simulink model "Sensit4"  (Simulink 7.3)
settings: Solver=ode45  StartTime=0.0  StopTime=10.0  RelTol=1e-3
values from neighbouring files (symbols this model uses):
  Kp3 = [0.3042  3.4539  0.5105  0.0711 -0.2670]    [run.m]
undefined symbols (not defined in the file or in its folder): Ap, Bp, Cp, Dp, TVC

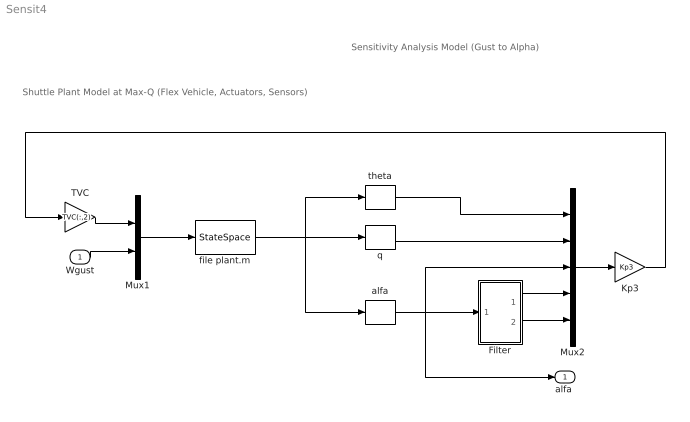
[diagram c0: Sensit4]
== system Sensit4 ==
  note: Shuttle Plant Model at Max-Q (Flex Vehicle, Actuators, Sensors)
  note: Sensitivity Analysis Model (Gust to Alpha)
  Wgust : Inport  OutDataType=sfix(16)  OutScaling=2^0
  Filter : Subsystem
  Kp3 : Gain  Gain=Kp3  Multiplication=Matrix(K*u)  ParameterDataType=sfix(16)  ParameterScaling=2^0  OutDataType=sfix(16)  OutScaling=2^0
  Mux1 : Mux  Inputs=[10,1]
  Mux2 : Mux  Inputs=5
  TVC : Gain  Gain=TVC(:,2)  Multiplication=Matrix(K*u)  ParameterDataType=sfix(16)  ParameterScaling=2^0  OutDataType=sfix(16)  OutScaling=2^0
  alfa : Selector  InputPortWidth=30  IndexOptions=Index vector (dialog)  Indices=[9]  OutputSizes=1
  file plant.m : StateSpace  A=Ap  B=Bp  C=Cp  D=Dp
  q : Selector  InputPortWidth=30  IndexOptions=Index vector (dialog)  Indices=[5]  OutputSizes=1
  theta : Selector  InputPortWidth=30  IndexOptions=Index vector (dialog)  Indices=[2]  OutputSizes=1
  "alfa " : Outport  OutDataType=sfix(16)  OutScaling=2^0
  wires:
  Mux2/1 -> Kp3/1
  Filter/1(x1) -> Mux2/4
  Filter/2(x2) -> Mux2/5
  theta/1 -> Mux2/1
  q/1 -> Mux2/2
  file plant.m/1 -> theta/1, q/1, alfa/1
  Mux1/1 -> file plant.m/1
  TVC/1 -> Mux1/1
  alfa/1 -> Filter/1(alfa), Mux2/3, "alfa "/1
  Wgust/1 -> Mux1/2
  Kp3/1 -> TVC/1

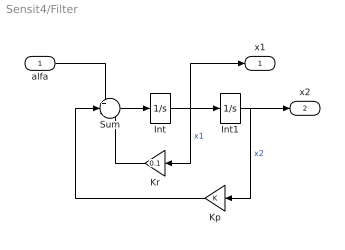
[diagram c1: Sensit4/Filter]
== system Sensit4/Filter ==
  alfa : Inport  OutDataType=sfix(16)  OutScaling=2^0
  Int : Integrator
  Int1 : Integrator
  Kp : Gain  ParameterDataType=sfix(16)  ParameterScaling=2^0  OutDataType=sfix(16)  OutScaling=2^0
  Kr : Gain  Gain=0.1  ParameterDataType=sfix(16)  ParameterScaling=2^0  OutDataType=sfix(16)  OutScaling=2^0
  Sum : Sum  Inputs=+--  OutDataType=sfix(16)  OutScaling=2^0
  x1 : Outport  OutDataType=sfix(16)  OutScaling=2^0
  x2 : Outport  Port=2  OutDataType=sfix(16)  OutScaling=2^0
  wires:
  Int/1 -> Int1/1, Kr/1, x1/1  "x1"
  Sum/1 -> Int/1
  Int1/1 -> Kp/1, x2/1  "x2"
  Kr/1 -> Sum/3
  Kp/1 -> Sum/2
  alfa/1 -> Sum/1
